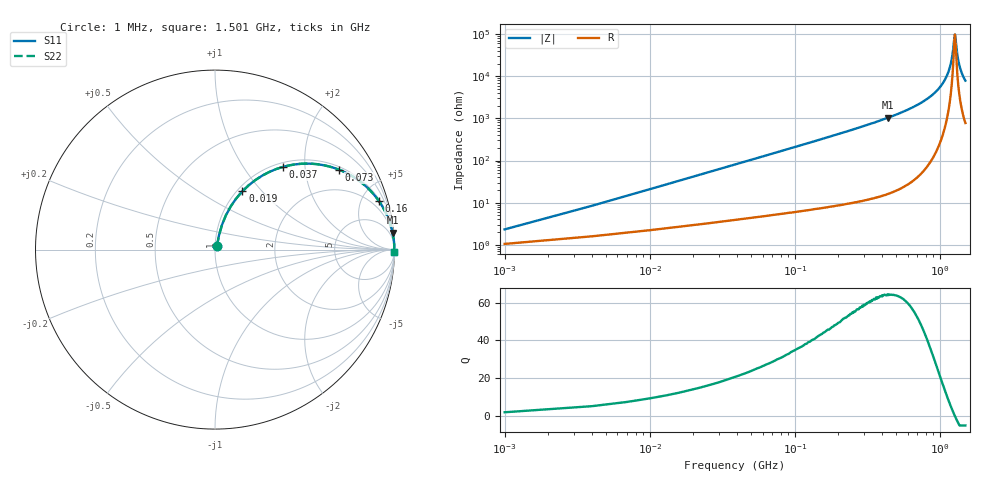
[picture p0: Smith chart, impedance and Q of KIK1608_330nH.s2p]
!version-2
!date-01.2022
!Series
# MHz S RI R 50
!Freq ReS11 ImS11 ReS21 ImS21 ReS12 ImS12 ReS22 ImS22
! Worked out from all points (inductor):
!   501 points, 1 MHz to 1.501 GHz, reference 50 ohm
!   read as one part in series: L = 330 nH near 7 MHz
!   highest Q = 64.2 at 442 MHz (marker M1), where L = 375 nH
!   self-resonance near 1.27 GHz
!   S11 on the Smith chart (normalised r, x): 1 MHz: 1.02, +0.04; 19 MHz: 1.06, +0.79; 37 MHz: 1.08, +1.54; 73 MHz: 1.10, +3.04; 160 MHz: 1.15, +6.74; 1.501 GHz: open
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1  0.0109 0.0203  0.9892 -0.0203  0.9892 -0.0203  0.0109 0.0203
10  0.0604 0.1906  0.9396 -0.1906  0.9396 -0.1906  0.0604 0.1906
19  0.1523 0.3247  0.8477 -0.3247  0.8477 -0.3247  0.1523 0.3247
37  0.3774 0.4605  0.6226 -0.4605  0.6226 -0.4605  0.3774 0.4605
73  0.6918 0.445  0.3082 -0.445  0.3082 -0.445  0.6918 0.445
109  0.8317 0.3606  0.1683 -0.3606  0.1683 -0.3606  0.8317 0.3606
160  0.9141 0.2692  0.0859 -0.2692  0.0859 -0.2692  0.9141 0.2692
253  0.9646 0.1759  0.0354 -0.1759  0.0354 -0.1759  0.9646 0.1759
442  0.9894 0.0947  0.0106 -0.0947  0.0106 -0.0947  0.9894 0.0947
502  0.9922 0.0803  0.00777 -0.0803  0.00777 -0.0803  0.9922 0.0803
751  0.9974 0.0416  0.00262 -0.0416  0.00262 -0.0416  0.9974 0.0416
1003  0.9988 0.0181  0.00119 -0.0181  0.00119 -0.0181  0.9988 0.0181
1099  0.999 0.011  0.00103 -0.011  0.00103 -0.011  0.999 0.011
1168  0.999 0.00637  0.000985 -0.00637  0.000985 -0.00637  0.999 0.00637
1216  0.999 0.00331  0.000989 -0.00331  0.000989 -0.00331  0.999 0.00331
1252  0.999 0.0011  0.00101 -0.0011  0.00101 -0.0011  0.999 0.0011
1264  0.999 0.000379  0.00102 -0.000379  0.00102 -0.000379  0.999 0.000379
1273  0.999 -0.000158  0.00102 0.000158  0.00102 0.000158  0.999 -0.000158
1315  0.9989 -0.00262  0.00107 0.00262  0.00107 0.00262  0.9989 -0.00262
1357  0.9989 -0.005  0.00112 0.005  0.00112 0.005  0.9989 -0.005
1420  0.9988 -0.00845  0.00124 0.00845  0.00124 0.00845  0.9988 -0.00845
1501  0.9986 -0.0126  0.00141 0.0126  0.00141 0.0126  0.9986 -0.0126
